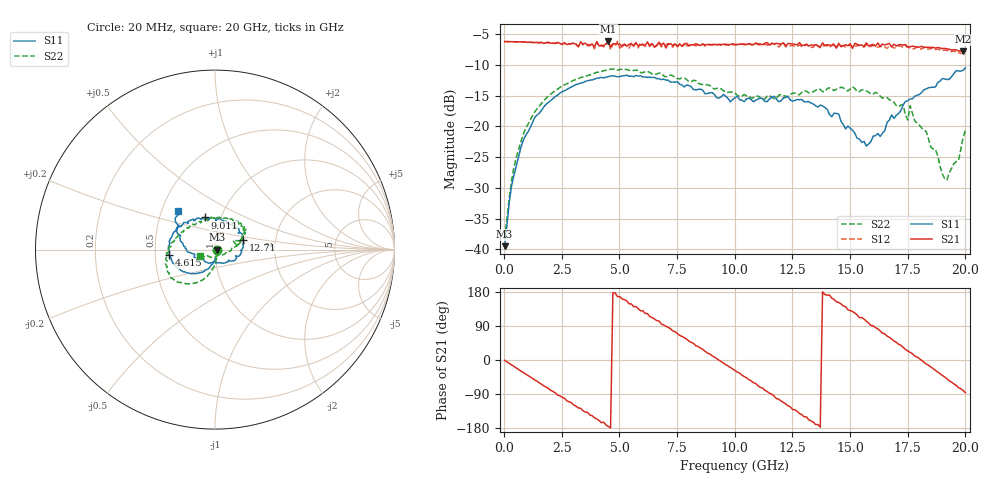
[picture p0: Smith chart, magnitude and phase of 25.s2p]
!Agilent Technologies,N5230A,US43500223,A.07.50.48
!Agilent N5230A: A.07.50.48
!Date: Tuesday, September 15, 2015 13:07:35
!Correction: S11(Full 2 Port(1,2))
!S21(Full 2 Port(1,2))
!S12(Full 2 Port(1,2))
!S22(Full 2 Port(1,2))
!S2P File: Measurements: S11, S21, S12, S22:
# Hz S  RI  R 50
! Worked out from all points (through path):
!   201 points, 20 MHz to 20 GHz, reference 50 ohm
!   highest |S21| = -6.17 dB at 4.516 GHz (marker M1); lowest = -7.8 dB at 19.9 GHz (marker M2)
!   group delay of S21, straight-line fit = 111 ps
!   lowest |S11| = -39.5 dB at 20 MHz (marker M3), VSWR 1.02, Z = 51.1 - j0.0696 ohm
!   |S11| at or under -10 dB: start of sweep to end of sweep
!   |S22| runs from -38.1 to -10.7 dB; largest |S21 - S12| = 0.052
!   S11 on the Smith chart (normalised r, x): 20 MHz: 1.02, -0.00; 4.615 GHz: 0.59, -0.04; 9.011 GHz: 0.84, +0.31; 12.71 GHz: 1.36, +0.14; 20 GHz: 0.61, +0.29
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2e7  0.0106 -0.000681  0.4889 -0.00664  0.4895 -0.00676  0.0123 -0.0015
3.197e8  0.00847 -0.0316  0.4755 -0.1085  0.4753 -0.1086  0.0129 -0.0337
9.191e8  -0.0164 -0.0824  0.3912 -0.2889  0.3887 -0.2899  -0.00604 -0.0949
2.3177e9  -0.1203 -0.1336  -0.0191 -0.4814  -0.0234 -0.4771  -0.0908 -0.1792
3.4166e9  -0.2001 -0.1066  -0.3226 -0.3367  -0.3354 -0.3161  -0.1661 -0.1894
4.5155e9  -0.2501 -0.0396  -0.4899 -0.0405  -0.4986 -0.0289  -0.2393 -0.159
4.6154e9  -0.2548 -0.0302  -0.4425 -0.00519  -0.4192 -0.00792  -0.2463 -0.1572
5.5145e9  -0.2552 0.0281  -0.4008 0.2487  -0.4149 0.2243  -0.2662 -0.0939
6.7133e9  -0.2193 0.1073  -0.1088 0.4712  -0.0932 0.4704  -0.2701 -0.022
7.9121e9  -0.1487 0.1579  0.2714 0.3886  0.2718 0.3605  -0.2371 0.041
9.011e9  -0.0581 0.1791  0.4537 0.0904  0.4526 0.0726  -0.1839 0.0992
1.001e10  0.0162 0.1698  0.4083 -0.218  0.3987 -0.2258  -0.1232 0.1411
1.14086e10  0.1061 0.1187  0.0552 -0.4768  0.032 -0.4598  -0.0278 0.1739
1.27073e10  0.1572 0.0514  -0.3271 -0.324  -0.3374 -0.2964  0.0733 0.166
1.34066e10  0.1517 0.00317  -0.4379 -0.1252  -0.4203 -0.125  0.1117 0.1552
1.43057e10  0.1217 -0.0392  -0.4338 0.1604  -0.4401 0.1771  0.1466 0.1289
1.57043e10  -0.003 -0.0691  -0.1023 0.4674  -0.0612 0.4565  0.1692 0.0944
1.67033e10  -0.1008 -0.0507  0.2374 0.4075  0.2437 0.3801  0.1504 0.0664
1.79021e10  -0.1766 0.0277  0.4393 0.0602  0.4394 0.033  0.1058 0.0147
1.92008e10  -0.1986 0.1349  0.2763 -0.3248  0.2484 -0.3332  0.012 -0.0345
1.99001e10  -0.2044 0.1989  0.0684 -0.4006  0.0442 -0.3959  -0.0706 -0.04
2e10  -0.2057 0.2177  0.0287 -0.4099  0.000276 -0.4008  -0.0856 -0.0355
